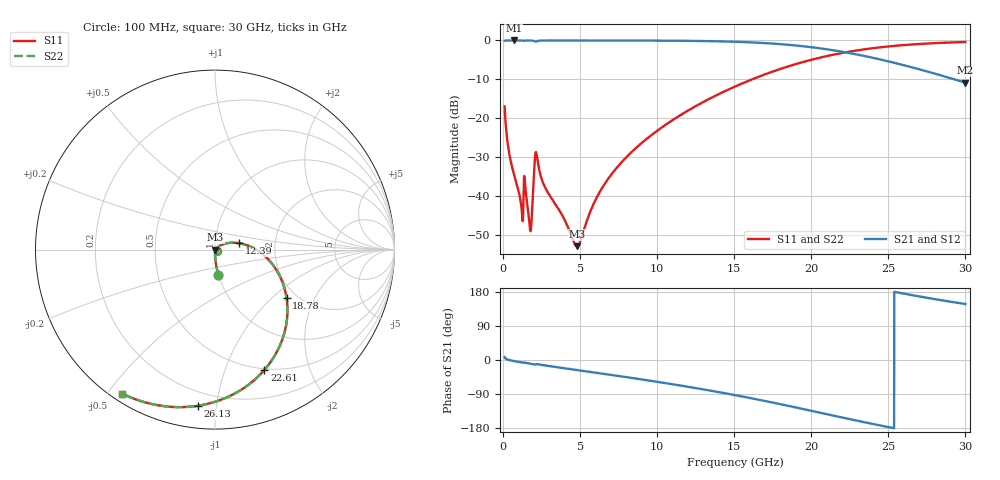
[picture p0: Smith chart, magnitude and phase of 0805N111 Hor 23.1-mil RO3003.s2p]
# GHz S MA R 50
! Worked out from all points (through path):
!   3201 points, 100 MHz to 30 GHz, reference 50 ohm
!   highest |S21| = -0.01 dB at 698 MHz (marker M1); lowest = -10.9 dB at 30 GHz (marker M2)
!   group delay of S21, straight-line fit = 20.5 ps
!   lowest |S11| = -52.9 dB at 4.791 GHz (marker M3), VSWR 1.00, Z = 50.2 - j0.106 ohm
!   |S11| at or under -10 dB: start of sweep to 16.17 GHz
!   |S22| runs from -52.9 to -0.4 dB; largest |S21 - S12| = 0
!   S11 on the Smith chart (normalised r, x): 100 MHz: 1.00, -0.29; 12.39 GHz: 1.30, +0.10; 18.78 GHz: 1.77, -1.24; 22.61 GHz: 0.49, -1.38; 26.13 GHz: 0.12, -0.89; 30 GHz: 0.03, -0.55
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0.1  0.1419 -82.3  0.9896 7.6  0.9896 7.6  0.1419 -82.3
0.3803125  0.03712 -89.2  0.9988 0.0  0.9988 0.0  0.03712 -89.2
0.698  0.01926 -90.7  0.9991 -2.8  0.9991 -2.8  0.01926 -90.7
1.165188  0.007849 -85.9  0.9985 -6.0  0.9985 -6.0  0.007849 -85.9
1.482875  0.01084 -81.1  0.9968 -7.6  0.9968 -7.6  0.01084 -81.1
1.753844  0.003684 -46.4  0.997 -9.6  0.997 -9.6  0.003684 -46.4
1.865969  0.005507 13.0  0.9949 -10.5  0.9949 -10.5  0.005507 13.0
2.071531  0.03101 -3.1  0.9693 -11.8  0.9693 -11.8  0.03101 -3.1
2.193  0.03271 -56.6  0.9768 -10.8  0.9768 -10.8  0.03271 -56.6
2.697563  0.01321 -89.8  0.9965 -14.2  0.9965 -14.2  0.01321 -89.8
4.790563  0.002252 -28.0  0.9976 -26.4  0.9976 -26.4  0.002252 -28.0
5.089563  0.002905 9.8  0.9975 -28.1  0.9975 -28.1  0.002905 9.8
6.836844  0.01675 42.8  0.997 -38.3  0.997 -38.3  0.01675 42.8
10.06978  0.07042 29.3  0.9938 -58.0  0.9938 -58.0  0.07042 29.3
12.38703  0.1385 15.0  0.9859 -73.3  0.9859 -73.3  0.1385 15.0
15.05  0.2549 -3.8  0.9614 -92.6  0.9614 -92.6  0.2549 -3.8
18.77816  0.4815 -34.1  0.8691 -123.3  0.8691 -123.3  0.4815 -34.1
20.03956  0.5659 -45.1  0.8166 -134.4  0.8166 -134.4  0.5659 -45.1
22.60909  0.7246 -67.7  0.6804 -157.0  0.6804 -157.0  0.7246 -67.7
25.01978  0.8374 -87.7  0.5369 -177.2  0.5369 -177.2  0.8374 -87.7
26.13169  0.8757 -96.4  0.4729 174.2  0.4729 174.2  0.8757 -96.4
30  0.9547 -122.8  0.2861 147.8  0.2861 147.8  0.9547 -122.8
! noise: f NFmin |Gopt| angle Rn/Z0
0.1  0.0003886  0.8463  0.6713  0.0005375
3.417  0.006687  0.7182  18.93  0.004571
6.743  0.009992  0.6499  36.73  0.004908
10.06  0.01381  0.636  53.46  0.005773
13.39  0.01813  0.6415  69.06  0.006633
16.7  0.0233  0.6598  83.47  0.007531
20.03  0.02991  0.6882  96.99  0.008544
23.35  0.03881  0.7252  109.8  0.009744
26.67  0.05159  0.7697  122.4  0.01118
30  0.07114  0.8189  135  0.01274
